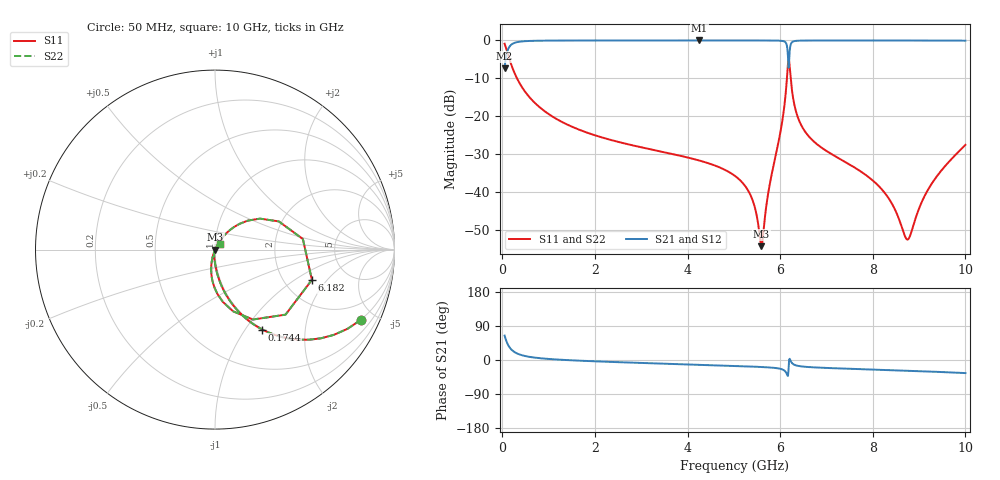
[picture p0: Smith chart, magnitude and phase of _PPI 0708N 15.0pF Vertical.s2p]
! S-Parameter data specifications (vertical orientation):
! Substrate: 40-mil Rogers 3003C, Substrate thickness, H=1.016mm, Dielectric constant, Er=3, Conductor thickness, T_mtl=0.043mm, Loss Tangent, Tand=0.003
! PCB Mounting Pad Footprint: Pad width, PadW=2.54mm , Pad length, PadL=0.51mm , Pad gap, PadG (edge-to-edge)=0.71mm , Reference planes=1.73mm apart
! Created Tue Jan 16 08:52:09 2018
# GHz S MA R 50
! 2 Port Network Data from SP1.SP block
! freq  magS11  angS11  magS21  angS21  magS12  angS12  magS22  angS22
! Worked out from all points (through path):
!   801 points, 50 MHz to 10 GHz, reference 50 ohm
!   highest |S21| = -0.01 dB at 4.254 GHz (marker M1); lowest = -7.4 dB at 50 MHz (marker M2)
!   group delay of S21, straight-line fit = 12.3 ps
!   lowest |S11| = -54.3 dB at 5.597 GHz (marker M3), VSWR 1.00, Z = 50.2 - j0.0669 ohm
!   |S11| at or under -10 dB: 316.9 MHz to 6.146 GHz (5.829 GHz wide, 180 % of centre); 6.227 GHz to end of sweep
!   |S22| runs from -54.3 to -0.9 dB; largest |S21 - S12| = 0
!   S11 on the Smith chart (normalised r, x): 50 MHz: 0.99, -4.19; 174.4 MHz: 0.99, -1.20; 6.182 GHz: 2.83, -1.40; 10 GHz: 1.06, +0.06
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0.05  0.9035 -25.5  0.4284 64.5  0.4284 64.5  0.9035 -25.5
0.174375  0.5176 -59.4  0.8554 30.6  0.8554 30.6  0.5176 -59.4
0.3360625  0.2999 -73.6  0.9537 16.3  0.9537 16.3  0.2999 -73.6
0.7091875  0.1483 -83.7  0.9885 6.2  0.9885 6.2  0.1483 -83.7
1.716625  0.06426 -91.5  0.9972 -2.1  0.9972 -2.1  0.06426 -91.5
3.370812  0.03469 -97.7  0.9983 -9.2  0.9983 -9.2  0.03469 -97.7
4.253875  0.02596 -100.3  0.9984 -12.6  0.9984 -12.6  0.02596 -100.3
5.025  0.01625 -101.0  0.9983 -15.7  0.9983 -15.7  0.01625 -101.0
5.37325  0.00869 -96.9  0.9982 -17.3  0.9982 -17.3  0.00869 -96.9
5.597125  0.001922 -20.3  0.9978 -18.5  0.9978 -18.5  0.001922 -20.3
5.77125  0.0122 58.1  0.9971 -19.7  0.9971 -19.7  0.0122 58.1
6.02  0.06911 59.0  0.9887 -23.8  0.9887 -23.8  0.06911 59.0
6.107062  0.1672 49.6  0.9547 -29.6  0.9547 -29.6  0.1672 49.6
6.181687  0.5656 -17.3  0.4359 -24.2  0.4359 -24.2  0.5656 -17.3
6.231438  0.2953 -81.4  0.894 -3.7  0.894 -3.7  0.2953 -81.4
6.281187  0.1708 -95.0  0.9678 -10.9  0.9678 -10.9  0.1708 -95.0
6.380687  0.09717 -102.5  0.99 -15.4  0.99 -15.4  0.09717 -102.5
6.691625  0.0485 -107.2  0.9968 -19.2  0.9968 -19.2  0.0485 -107.2
8.345812  0.008185 -102.8  0.9977 -26.7  0.9977 -26.7  0.008185 -102.8
8.768688  0.002382 -21.9  0.9973 -28.5  0.9973 -28.5  0.002382 -21.9
9.241312  0.01199 44.0  0.9964 -30.6  0.9964 -30.6  0.01199 44.0
10  0.04181 45.1  0.9912 -34.6  0.9912 -34.6  0.04181 45.1
